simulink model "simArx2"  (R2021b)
settings: Solver=VariableStepAuto  StartTime=0.0  StopTime=zt.SamplingInstants(end)  RelTol=1e-3
libraries: slident x1, cstblocks x1

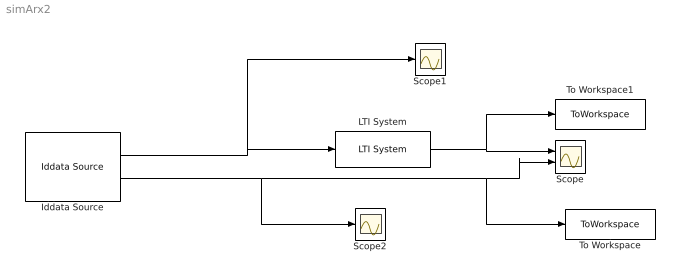
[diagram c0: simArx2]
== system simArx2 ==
  Iddata Source : slident/Iddata Source  iddataobj=zt
  LTI System : cstblocks/LTI System  sys=full_miso_model  IC=[]
  Scope : Scope  NumInputPorts=2
  Scope1 : Scope
  Scope2 : Scope
  To Workspace : ToWorkspace  VariableName=y  SampleTime=-1
  To Workspace1 : ToWorkspace  VariableName=sim_y  SampleTime=-1
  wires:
  Iddata Source/1 -> Scope1/1, LTI System/1
  Iddata Source/2 -> Scope2/1, To Workspace/1, Scope/2
  LTI System/1 -> To Workspace1/1, Scope/1
